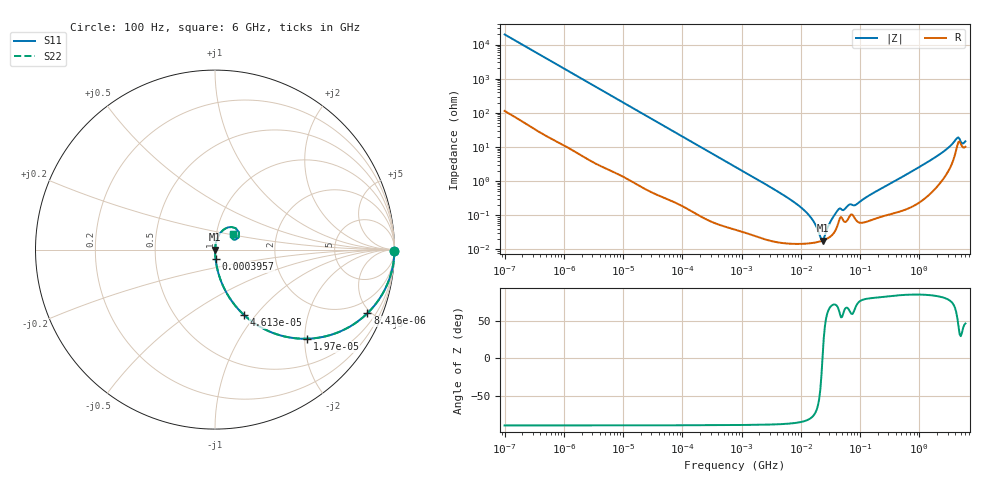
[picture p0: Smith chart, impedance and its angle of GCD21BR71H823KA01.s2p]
!Murata Part Number: GCD21BR71H823KA01
!These Parameters are Measured in Series Mode Connection
!Data Generated on Mar 13, 2026
!  o--ll--o
!Port1  Port2
!  o------o
!Operation Temp=25[degC], DC Bias Voltage=0[V]
!Freq. Start=100[Hz] Stop=6[GHz] 401[Steps]
# Hz S RI R 50
!Freq.(Hz) S11(Real) S11(Imag) S21(Real) S21(Imag) S12(Real) S12(Imag) S22(Real) S22(Imag)
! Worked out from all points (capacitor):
!   401 points, 100 Hz to 6 GHz, reference 50 ohm
!   read as one part in series: C = 80.2 nF near 109 Hz
!   lowest |Z| = 18 mohm at 23.28 MHz (marker M1)
!   series resonance near 23.2 MHz, so ESL is about 590 pH
!   S11 on the Smith chart (normalised r, x): 100 Hz: open; 8.416 kHz: 1.03, -4.78; 19.7 kHz: 1.01, -2.05; 46.13 kHz: 1.01, -0.88; 395.7 kHz: 1.00, -0.10; 6 GHz: 1.20, +0.21
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100  0.9999 -0.00505  5.45e-05 0.00505  5.45e-05 0.00505  0.9999 -0.00505
2008  0.9895 -0.0992  0.0105 0.0992  0.0105 0.0992  0.9895 -0.0992
8416  0.8494 -0.3544  0.1506 0.3544  0.1506 0.3544  0.8494 -0.3544
19704  0.512 -0.4965  0.488 0.4965  0.488 0.4965  0.512 -0.4965
40335  0.203 -0.3985  0.797 0.3985  0.797 0.3985  0.203 -0.3985
46134  0.1635 -0.366  0.8365 0.366  0.8365 0.366  0.1635 -0.366
103284  0.039 -0.189  0.961 0.189  0.961 0.189  0.039 -0.189
395726  0.00321 -0.0515  0.9968 0.0515  0.9968 0.0515  0.00321 -0.0515
774597  0.00108 -0.0265  0.9989 0.0265  0.9989 0.0265  0.00108 -0.0265
6948629  0.000153 -0.00273  0.9998 0.00273  0.9998 0.00273  0.000153 -0.00273
1.137099e7  0.000148 -0.0014  0.9999 0.0014  0.9999 0.0014  0.000148 -0.0014
1.555665e7  0.000154 -0.000745  0.9998 0.000745  0.9998 0.000745  0.000154 -0.000745
2.128304e7  0.000171 -0.000159  0.9998 0.000159  0.9998 0.000159  0.000171 -0.000159
2.327686e7  0.00018 5.9e-06  0.9998 -5.9e-06  0.9998 -5.9e-06  0.00018 5.9e-06
2.545746e7  0.000191 0.000173  0.9998 -0.000173  0.9998 -0.000173  0.000191 0.000173
3.330331e7  0.000257 0.000715  0.9997 -0.000715  0.9997 -0.000715  0.000257 0.000715
4.35672e7  0.000641 0.00136  0.9994 -0.00136  0.9994 -0.00136  0.000641 0.00136
8.527865e7  0.000725 0.0019  0.9993 -0.0019  0.9993 -0.0019  0.000725 0.0019
3.124326e8  0.00112 0.0081  0.9989 -0.0081  0.9989 -0.0081  0.00112 0.0081
1.95892e9  0.00926 0.0518  0.9907 -0.0518  0.9907 -0.0518  0.00926 0.0518
4.193612e9  0.0923 0.1259  0.9077 -0.1259  0.9077 -0.1259  0.0923 0.1259
6e9  0.1006 0.0866  0.8994 -0.0866  0.8994 -0.0866  0.1006 0.0866
